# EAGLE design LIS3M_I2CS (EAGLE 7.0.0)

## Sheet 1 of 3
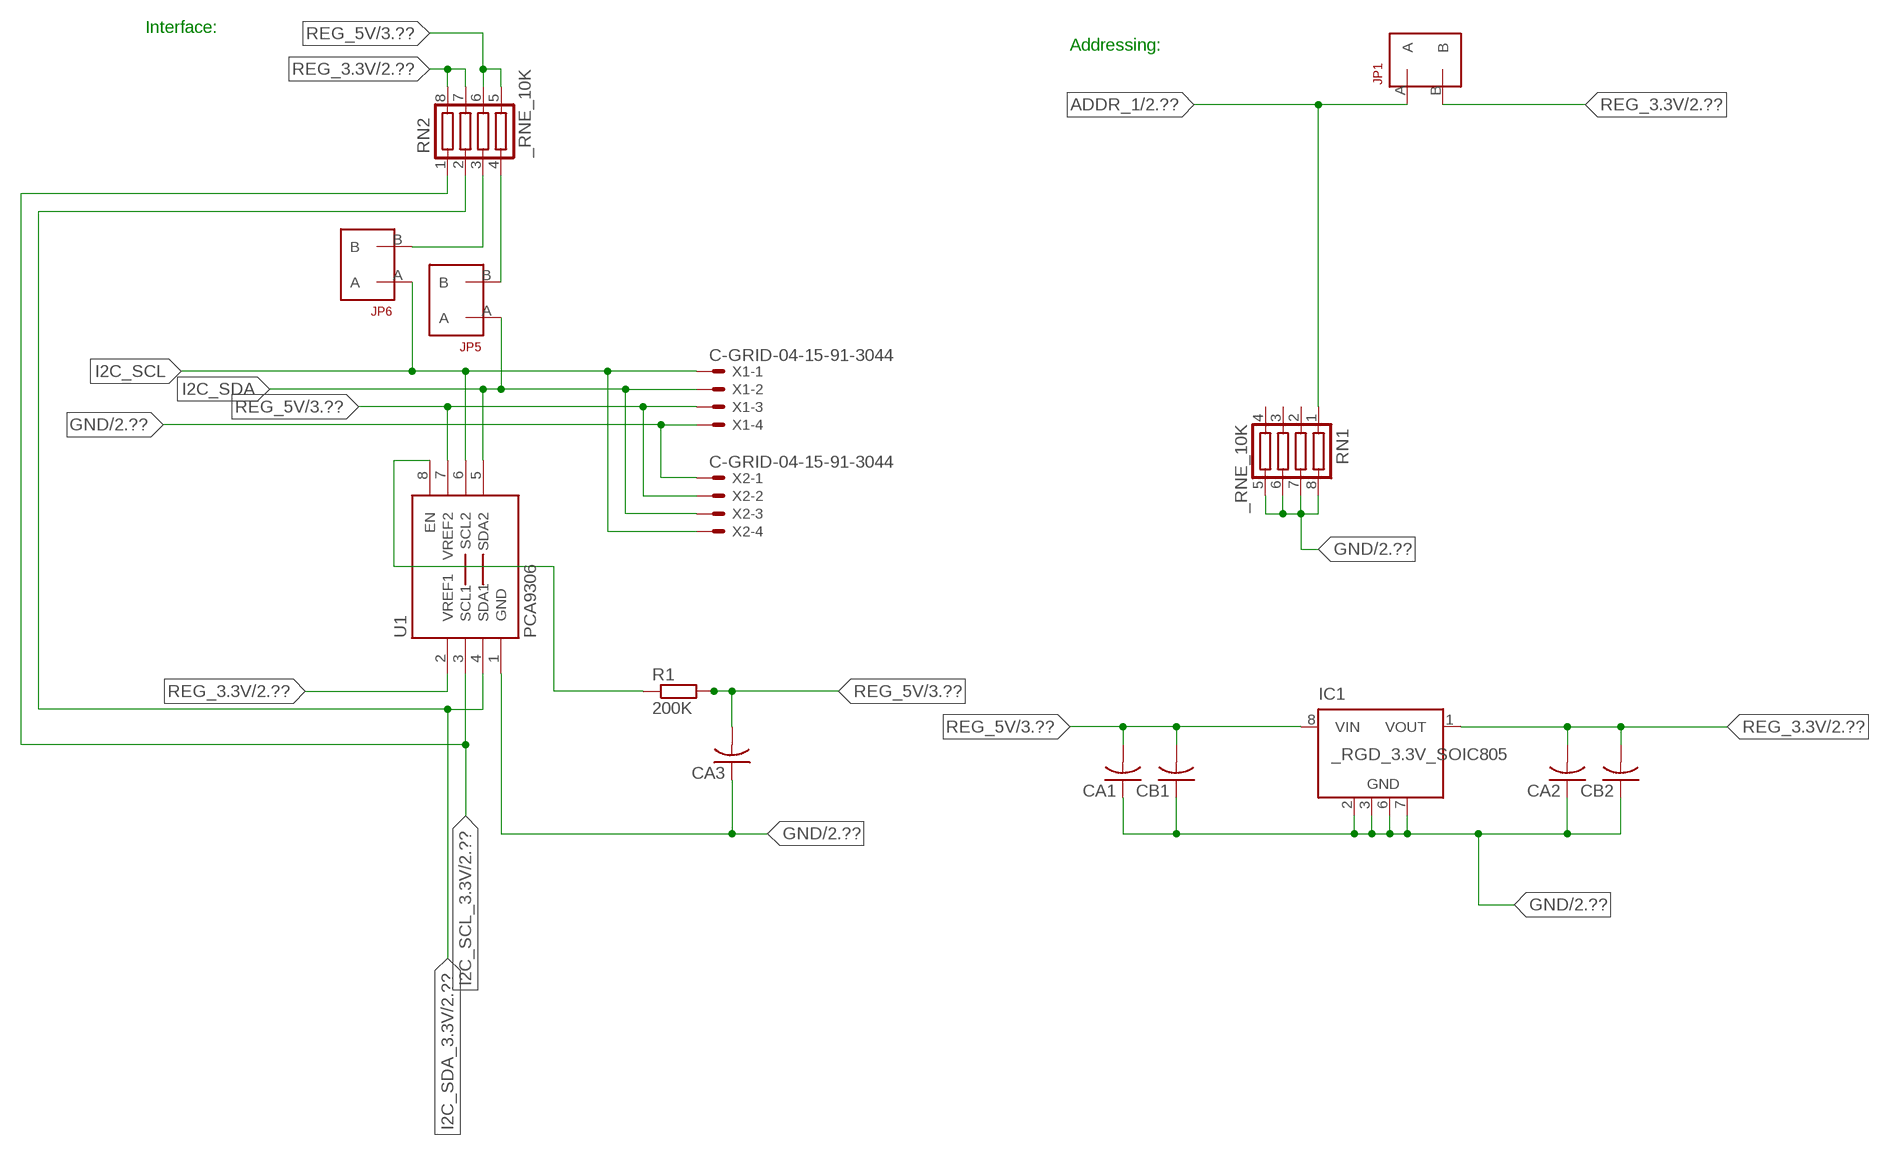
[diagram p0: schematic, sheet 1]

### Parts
CA1  CC1206KRX7R9BB104  [.1UF]
CA2  CC1206KRX7R9BB104  [.1UF]
CA3  CC1206KRX7R9BB104  [.1UF]
CB1  TMK316F106ZL-TC1206K  [TMK316F106ZL-T]
CB2  TMK316F106ZL-TC1206K  [TMK316F106ZL-T]
IC1  _RGD_3.3V_SOIC805  [_RGC_3.3V_SOIC8]
JP1  JUMPER_1X2_2MM  [JUMPER_1X2_2MM]
JP5  JUMPER_1X2_2MM  [JUMPER_1X2_2MM]
JP6  JUMPER_1X2_2MM  [JUMPER_1X2_2MM]
R1  200K  RESISTOR_SMT-0603  [R603]
RN1  _RNE_10K  [RNE]
RN2  _RNE_10K  [RNE]
U1  PCA9306  PCA9306_NCD  [PSOP-8]
X1  C-GRID-04-15-91-3044  [15-91-04]
X2  C-GRID-04-15-91-3044  [15-91-04]

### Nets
ADDR_1: JP1.A RN1.1 ; also sheet 2
GND: CA1.1 CA2.1 CA3.1 CB1.1 CB2.1 IC1.2(GND) IC1.3(GND) IC1.6(GND) IC1.7(GND) RN1.5 RN1.6 RN1.7 RN1.8 U1.1(GND) X1.4 X2.1 ; also sheet 2,3
I2C_SCL: JP6.A U1.6(SCL2) X1.1 X2.4
I2C_SCL_3.3V: RN2.1 U1.3(SCL1) ; also sheet 2
I2C_SDA: JP5.A U1.5(SDA2) X1.2 X2.3
I2C_SDA_3.3V: RN2.2 U1.4(SDA1) ; also sheet 2
N$1: JP6.B RN2.3
N$2: JP5.B RN2.4
N$23: R1.1 U1.8(EN)
REG_3.3V: CA2.2 CB2.2 IC1.1(VOUT) JP1.B RN2.7 RN2.8 U1.2(VREF1) ; also sheet 2
REG_5V: CA1.2 CA3.2 CB1.2 IC1.8(VIN) R1.2 RN2.5 RN2.6 U1.7(VREF2) X1.3 X2.2 ; also sheet 3
Unconnected: IC1.4(NC) IC1.5(NC) RN1.2 RN1.3 RN1.4

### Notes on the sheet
- Interface:
- Addressing:

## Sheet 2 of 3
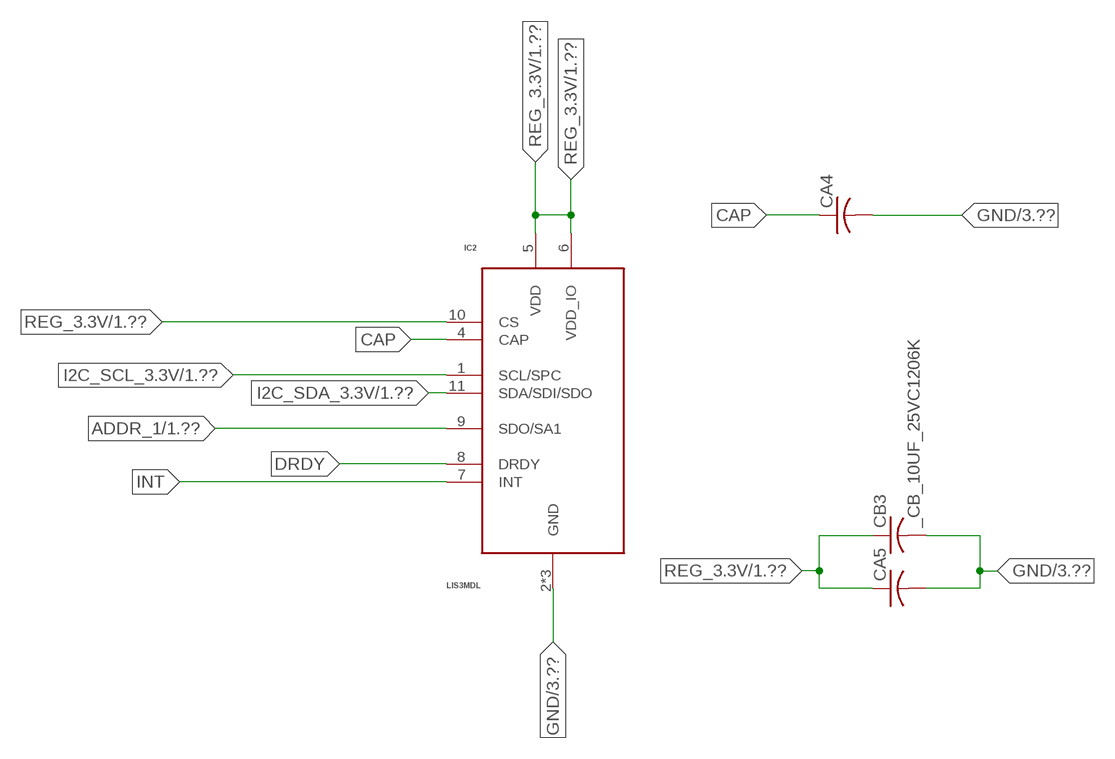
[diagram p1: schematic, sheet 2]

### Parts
CA4  _CA_.10UF_50VC1206K  [_CA_.1UF_50V]
CA5  _CA_.10UF_50VC1206K  [_CA_.1UF_50V]
CB3  _CB_10UF_25VC1206K  [_CB_10UF_25V]
IC2  LIS3MDL  [LGA-12]

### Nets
ADDR_1: IC2.9(SDO/SA1) ; also sheet 1
CAP: CA4.1 IC2.4(CAP)
DRDY: IC2.8(DRDY)
GND: CA4.2 CA5.2 CB3.2 IC2.2(GND) IC2.3(GND) IC2.12(GND) ; also sheet 1,3
I2C_SCL_3.3V: IC2.1(SCL/SPC) ; also sheet 1
I2C_SDA_3.3V: IC2.11(SDA/SDI/SDO) ; also sheet 1
INT: IC2.7(INT)
REG_3.3V: CA5.1 CB3.1 IC2.5(VDD) IC2.6(VDD_IO) IC2.10(CS) ; also sheet 1

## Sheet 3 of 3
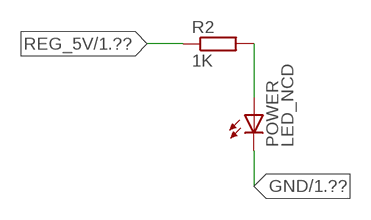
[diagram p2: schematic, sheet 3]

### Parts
POWER  LED_NCD  [CHIPLED_0603]
R2  1K  RESISTOR_SMT-0402  [R402]

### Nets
GND: POWER.C ; also sheet 1,2
N$4: POWER.A R2.2
REG_5V: R2.1 ; also sheet 1

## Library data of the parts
CA1-CA3 = NCD_ULTIMATE_LIBRARY:CC1206KRX7R9BB104: Capacitor CA .1uF 50V SMT C1206K CC1206KRX7R9BB104
CA4 CA5 = NCD_ULTIMATE_LIBRARY:_CA_.10UF_50V: Capacitor .1uF SMT
CB1 CB2 = NCD_ULTIMATE_LIBRARY:TMK316F106ZL-T: Capacitor CB 10uF SMT 1206 TMK316F106ZL-T
CB3 = NCD_ULTIMATE_LIBRARY:_CB_10UF_25V: Capacitor 10uF SMT
IC1 = NCD_ULTIMATE_LIBRARY:_RGD_3.3V_SOIC8: Regulator Linear 3.3V Chip Positive VOLTAGE REGULATOR Digikey 497-1199-2-ND/L78L33ACD13TR
IC2 = NCD_ULTIMATE_bhaskar:LIS3MDL: Digikey 497-13892-6-ND/LIS3MDLTR
JP1 JP5 JP6 = NCD_ULTIMATE_CONNECTORS:JUMPER_1X2_2MM
POWER = NCD_ULTIMATE_LIBRARY:LED_NCD: LED Digikey 754-1132-2-ND/APT2012SRCPRV
R1 R2 = NCD_ULTIMATE_LIBRARY:RESISTOR_SMT: NCD Resistor
RN1 RN2 = NCD_ULTIMATE_LIBRARY:_RNE_10K: Resistor Array RNE SMT 10K x 4 Single Resistor Source: http://www.ctscorp.com/components/Datasheets/CTSChipArrayDs.pdf Digikey 742C083103JPTR-ND/742C083103JP; OC_FARNELL: unknown; OC_NEWARK: unknown
U1 = NCD_ULTIMATE_LIBRARY:PCA9306_NCD: NCD Bidirectional I2C level shifter. NOT compatible with all available part number pinout schemes- DOUBLE CHECK!!!; PROD_ID: IC-10023
X1 X2 = NCD_ULTIMATE_CONNECTORS:C-GRID-04: CONNECTOR 4-Pos I2C wire to board 2.54 mm (0.100") pitch header Digikey WM1342-ND/0015912045; OC_FARNELL: unknown; OC_NEWARK: unknown

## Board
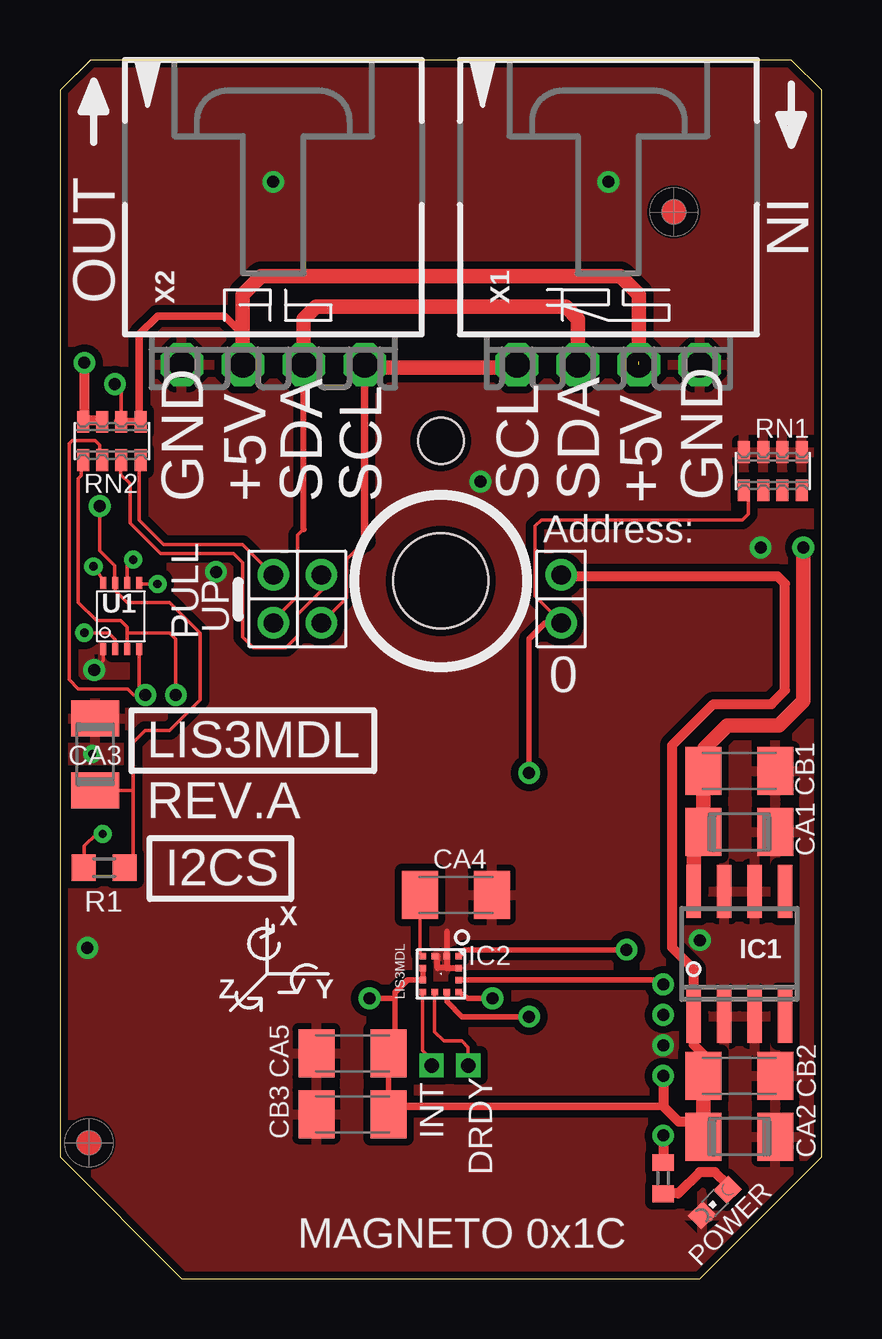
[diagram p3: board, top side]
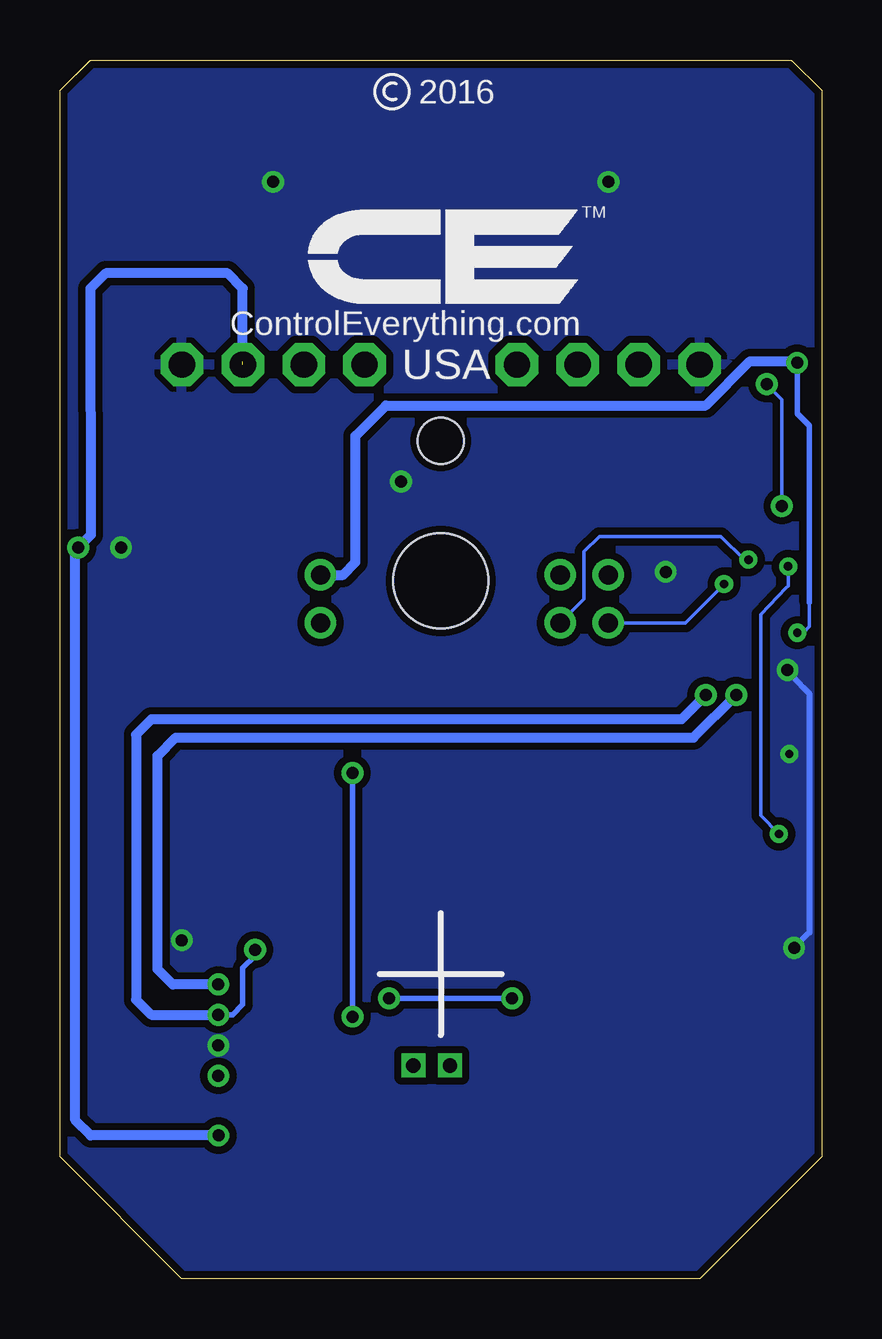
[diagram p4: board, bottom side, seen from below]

Size 31.75 x 50.8 mm. Coordinates in mm from the lower left corner, seen from the top.
Outline: 32 segments
Copper layers (1*16): Top 0.035mm / dielectric 1.5mm / Bottom 0.035mm
Design rules "default": minimum track width 5mil, minimum drill 24mil, track to track 5mil, track to pad 5mil, pad to pad 5mil, via to via 5mil, smd to smd 5mil, copper to edge 10mil, drill to drill 8mil, minimum pad ring 10mil, minimum via ring 8mil, stop-mask expansion 2mil, vias tented up to drill 0mil, thermal gap 10mil
Holes 3.96 mm at 15.88,29.08
Holes 1.91 mm at 15.88,34.93

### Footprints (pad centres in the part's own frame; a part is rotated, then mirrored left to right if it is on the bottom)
.1UF = smd 1.5 x 2: 1 -1.5,0; 2 1.5,0
_CA_.1UF_50V = smd 1.5 x 2: 1 -1.5,0; 2 1.5,0
TMK316F106ZL-T = smd 1.5 x 2: 1 -1.5,0; 2 1.5,0
_CB_10UF_25V = smd 1.5 x 2: 1 -1.5,0; 2 1.5,0
_RGC_3.3V_SOIC8 = smd 0.6 x 2.2: 1 -1.905,-2.6; 2 -0.635,-2.6; 3 0.635,-2.6; 4 1.905,-2.6; 5 1.905,2.6; 6 0.635,2.6; 7 -0.635,2.6; 8 -1.905,2.6
LGA-12 = smd 0.275 x 0.275: 1 -0.75,0.75; 2 -0.75,0.25; 3 -0.75,-0.25; 4 -0.75,-0.75; 5 -0.25,-0.75; 6 0.25,-0.75; 7 0.75,-0.75; 8 0.75,-0.25; 9 0.75,0.25; 10 0.75,0.75; 11 0.25,0.75; 12 -0.25,0.75
JUMPER_1X2_2MM = drill 0.8: A 0,2; B 0,0
CHIPLED_0603 = smd 0.8 x 0.876: A 0,-0.75; C 0,0.75
R603 = smd 1 x 1.1: 1 -0.85,0; 2 0.85,0
R402 = smd 0.7 x 0.9: 1 -0.65,0; 2 0.65,0
RNE = smd 0.5 x 0.9: 1 -1.2,-0.8; 2 -0.4,-0.8; 3 0.4,-0.8; 4 1.2,-0.8; 5 1.2,0.8; 6 0.4,0.8; 7 -0.4,0.8; 8 -1.2,0.8
PSOP-8 = smd 0.25 x 0.5: 1 -0.73,-1.37; 2 -0.23,-1.37; 3 0.27,-1.37; 4 0.77,-1.37; 5 0.77,1.38; 6 0.27,1.38; 7 -0.23,1.38; 8 -0.73,1.38
15-91-04 = drill 1.1 pad 1.778 octagon: 1 -3.81,-7.62; 2 -1.27,-7.62; 3 1.27,-7.62; 4 3.81,-7.62

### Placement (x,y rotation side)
CA1  28.32,18.62 180 top
CA2  28.32,5.92 180 top
CA3  1.46,21.86 270 top
CA4  16.51,16 0 top
CA5  12.19,9.4 180 top
CB1  28.32,21.16 180 top
CB2  28.32,8.46 180 top
CB3  12.19,6.86 180 top
IC1  28.32,13.54 0 top
IC2  15.88,12.7 270 top
JP1  20.89,29.34 180 top
JP5  8.89,29.34 180 top
JP6  10.9,29.34 180 top
POWER  27.3,3.18 135 top
R1  1.84,17.13 0 top
R2  25.15,4.19 270 top
RN1  29.72,33.66 0 top
RN2  2.16,34.93 0 top
U1  2.54,27.61 0 top
U$5  [VISION_REF10]  1.21,5.66 90 top
U$28  [VISION_REF10]  25.59,44.46 90 top
X1  22.86,45.72 0 top
X2  8.89,45.72 0 top

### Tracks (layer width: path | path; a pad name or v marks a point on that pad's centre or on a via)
ADDR_1  (via drill 0.5)
  Top 0.152: JP1.A 20.89,27.37 19.81,28.45 19.81,31.37 20.07,31.62 28.45,31.62 28.7,31.88 28.7,32.78 RN1.1
  Top 0.229: IC2.9 16.13,11.56 16.76,10.92 v19.56,10.92 | v19.56,21.08 19.56,26.67 20.23,27.34 JP1.A
  Bottom 0.229: v19.56,10.92 v19.56,21.08
CAP
  Top 0.152: IC2.4 15.01,13.57 CA4.1
DRDY  (via drill 0.6)
  Top 0.152: IC2.8 15.62,10.29 16,9.91 16.76,9.91 17.02,9.65 v17.02,8.89
GND  (via drill 0.35, 0.5)
  Top 0.152: CA3.1 1.52,23.42 1.52,23.62 | v1.42,25.38 1.81,25.76 U1.1
  Top 0.229: 16.13,14.48 16.13,13.58 IC2.2
  Top 0.254: IC2.2 16.12,12.96 16.13,12.95 | 16.13,12.95 IC2.12 | 16.13,13.58 16.13,12.95 | 16.13,12.95 15.75,12.95 15.75,13.45 IC2.3
  Bottom 0.254: v1.42,25.38 0.76,24.64 0.51,24.38 0.51,14.43 v1.15,13.79
  other vias: 8.89,45.72 22.86,45.72 25.15,9.73 17.53,33.22 26.67,14.11 6.5,29.46 29.21,30.48 1.35,21.87
  pour Bottom (isolate 0.305): -0.64,5.08 -0.64,49.53 1.27,51.44 30.48,51.44 32.38,49.53 32.38,5.08 26.67,-0.63 5.08,-0.63
  pour Top (isolate 0.305): 4.45,-1.27 -1.27,4.45 -1.27,50.17 0.64,52.07 31.11,52.07 33.02,50.17 33.02,4.45 27.3,-1.27
I2C_SCL  (via drill 0.35)
  Top 0.152: 12.7,30.73 11.94,29.97 11.94,28.38 JP6.A | v3.05,29.97 2.81,29.73 U1.6
  Top 0.305: 12.7,30.73 X2.4
  Top 0.406: X2.4 12.7,37.97 | 19.05,37.97 X1.1
  Top 0.61: 12.7,37.97 19.05,37.97
  Bottom 0.152: JP6.A 9.91,28.33 9.91,30.3 9.27,30.94 4.19,30.94 3.23,29.97 v3.05,29.97
I2C_SCL_3.3V  (via drill 0.5)
  Top 0.152: RN2.1 0.89,34.07 0.89,33.48 0.77,33.35 0.77,28.59 0.76,28.59 0.76,28.19 1.52,27.43 2.54,27.43 2.81,27.17 2.81,26.92 | 2.81,26.92 U1.3 | v4.83,24.33 v4.83,24.34 4.83,26.67 4.57,26.92 2.81,26.92
  Top 0.229: v23.62,13.72 16.89,13.72 IC2.1
  Bottom 0.229: v25.15,11 24.56,11 24.13,11.43 24.13,12.95 23.62,13.46 v23.62,13.72
  Bottom 0.406: v4.83,24.33 5.84,23.32 27.94,23.32 28.58,22.68 28.58,11.63 27.94,11 v25.15,11
I2C_SDA  (via drill 0.35)
  Top 0.152: JP5.A 8.89,27.44 9.91,28.45 9.91,30.99 10.16,31.24 | U1.5 3.34,28.96 v4.06,28.96
  Top 0.254: 10.16,31.24 10.16,31.25 X2.3
  Top 0.61: X2.3 10.16,40.01 10.67,40.51 21.09,40.51 21.59,40.01 X1.2
  Bottom 0.152: v4.06,28.96 5.68,27.34 JP5.A
I2C_SDA_3.3V  (via drill 0.5)
  Top 0.152: RN2.2 1.65,34.14 1.65,34.75 1.46,34.94 0.51,34.94 0.38,34.81 0.38,26.37 0.38,26.36 0.38,24.97 0.76,24.59 2.82,24.59 3.07,24.33 v3.56,24.33 3.31,24.58 U1.4
  Top 0.229: IC2.11 16.76,12.45 24.97,12.45 v25.15,12.27
  Bottom 0.406: v25.15,12.27 27.05,12.27 27.69,12.9 27.69,21.79 26.93,22.56 5.34,22.56 v3.56,24.33
INT  (via drill 0.6)
  Top 0.152: IC2.7 15.11,11.81 15.11,9.53 15.49,9.14 v15.49,8.89
N$1
  Top 0.152: JP6.B 10.92,29.31 10.92,28.7 9.91,27.69 9.91,26.8 9.42,26.31 8.06,26.31 7.62,26.75 7.62,29.84 7.24,30.23 4.19,30.23 2.92,31.5 2.92,33.15 2.54,33.53 2.54,34.1 RN2.3
  Top 0.305: 2.54,34.02 RN2.3
N$2
  Top 0.152: JP5.B 7.62,30.61 4.32,30.61 3.3,31.62 3.3,34.07 RN2.4
  Top 0.305: 3.37,33.88 RN2.4
N$4
  Top 0.406: POWER.A 27.84,3.92 27.3,4.45 26.67,4.45 25.78,3.56 25.16,3.56 R2.2
N$23  (via drill 0.35)
  Top 0.152: R1.1 1.02,17.16 1.02,18.03 1.52,18.54 v1.78,18.54 | v1.4,29.69 1.81,29.13 U1.8
  Bottom 0.152: v1.78,18.54 2.54,19.3 2.54,27.69 1.47,28.8 1.4,28.88 v1.4,29.69
REG_3.3V  (via drill 0.35, 0.5)
  Top 0.152: v1.02,26.92 2.03,26.92 2.31,26.65 U1.2
  Top 0.229: 13.72,6.83 CB3.1 CA5.1 13.97,10.14 13.97,11.68 | 26.42,5.08 26.82,5.49 CA2.2 | 13.97,11.68 13.97,11.94 14.48,12.45 IC2.6 IC2.5 | v12.9,11.68 13.97,11.68 | IC2.10 17.02,11.68 v18.03,11.68
  Top 0.305: 13.72,6.83 14.07,7.19 25.15,7.19
  Top 0.406: CB2.2 26.82,9.35 26.42,9.75 26.42,10.36 | v25.15,8.46 25.15,7.19 25.78,6.55 26.82,6.55 | IC1.1 26.42,12.9 25.53,13.79 25.53,22.24 27.24,23.95 29.66,23.95 30.23,24.52 30.23,28.97 29.91,29.29 20.95,29.29 JP1.B | 26.52,5.62 CA2.2 | v1.02,38.18 1.02,35.78 | 1.02,35.78 RN2.8 | 1.02,35.78 1.71,35.78 RN2.7
  Top 0.61: CB2.2 26.82,6.55 CA2.2 | 26.42,10.36 IC1.1
  Bottom 0.152: 0.51,28.19 0.51,27.18 0.76,26.92 v1.02,26.92
  Bottom 0.229: 0.51,28.19 0.51,35.56 1.02,36.07 v1.02,38.18 | v18.03,11.68 v12.9,11.68
  Bottom 0.406: v1.02,38.18 1.08,38.24 2.99,38.24 4.83,36.4 18.16,36.4 19.43,35.13 19.43,29.87 19.94,29.34 JP1.B
REG_5V  (via drill 0.5)  (1 unrouted)
  Top 0.152: RN2.6 2.56,37.01 v2.29,37.29 | R1.2 3.05,17.49 3.05,20.36 | 3.05,20.36 3.05,22.35 3.56,22.86 4.57,22.86 5.84,24.13 5.84,26.92 4.57,28.19 2.79,28.19 2.31,28.68 U1.7 2.29,29.01 2.29,29.72 1.65,30.35 v1.65,32.21 | CA3.2 3.05,20.36
  Top 0.305: 7.62,39.37 7.5,39.37 | 2.42,35.74 RN2.6 RN2.5 3.31,35.8 3.31,39.37 4.07,40.13 6.86,40.13 7.62,39.37 | X2.2 7.62,39.37
  Top 0.406: v25.15,5.97 R2.1
  Top 0.61: X2.2 7.62,41.02 8.38,41.78 23.37,41.78 24.13,41.02 X1.3 | IC1.8 26.42,18.21 CA1.2 CB1.2 26.86,21.2 26.86,22.11 27.82,23.06 29.98,23.06 30.99,24.08 v30.99,30.48
  Bottom 0.152: v1.65,32.21 1.65,36.65 v2.29,37.29
  Bottom 0.406: 24.13,38.23 24.13,41.28 24.77,41.91 29.84,41.91 30.48,41.27 30.47,31 v30.99,30.48 31.11,30.36 31.11,6.6 30.48,5.97 v25.15,5.97

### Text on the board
tPlace: X | Z | Y
tNames: IN | OUT | GND | +5V | SDA | SCL | SCL | SDA | +5V | GND | Address: | PULL | UP | 0 | LIS3MDL | REV.A | I2CS | INT | DRDY | MAGNETO 0x1C
bNames: 2016 | TM | ControlEverything.com | USA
